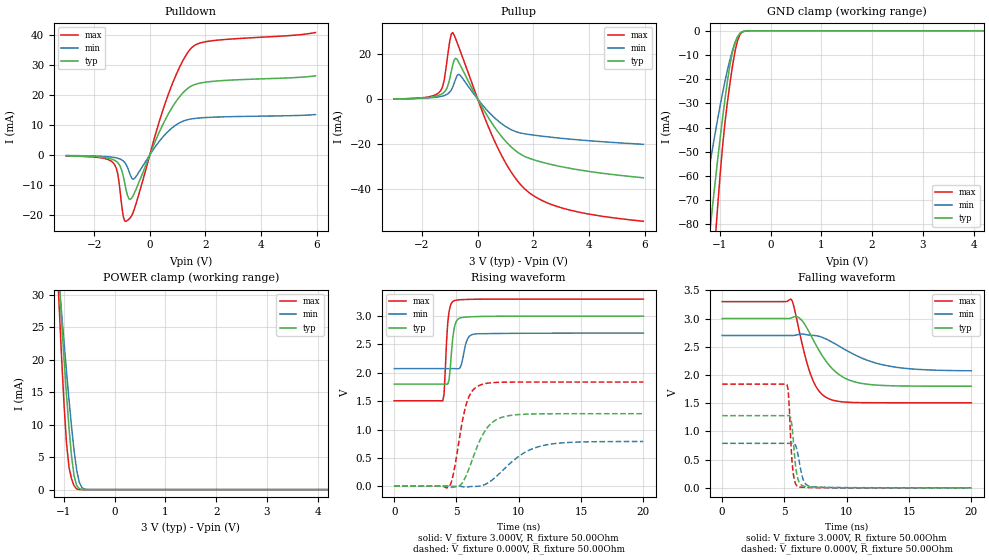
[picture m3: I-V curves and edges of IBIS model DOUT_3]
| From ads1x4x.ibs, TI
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|   DOutput 3.0V Model
[Model]   DOUT_3
Model_type   3-state
|Signals   DOUT_nDRDY
| variable   typ   min   max
|C_comp Output Tri-state
C_comp   3.796pF   4.715pF   2.919pF
|C_comp Output Low
|C_comp   7.402pF   8.505pF   5.981pF
|C_comp Output High
|C_comp   7.018pF   8.098pF   7.325pF
[Model Spec]
|Timing spec test load voltage corners 0.45*VCC
Vmeas   1.5V   1.35V   1.65V
Vref   1.5V   1.35V   1.65V
|Junction Temperature
[Temperature Range]   40.0   105.0   -40.0
[Voltage range]   5.0V   4.75V   5.25V
[Pullup reference]   3.0V   2.7V   3.3V
[power clamp reference]   3.0V   2.7V   3.3V
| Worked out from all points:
|   slope of the pulldown table from 0 to 0.45 V, typ, clamps not added: 45.9 ohm
|   slope of the pullup table from 0 to 0.45 V, typ, clamps not added: 47.3 ohm
|   GND clamp passes 1 mA (typ) near -0.60 V on its own axis
|   POWER clamp passes 1 mA (typ) near -0.76 V on its own axis
|   falling waveform, V_fixture 3.000V, R_fixture 50.00Ohm: 20-80 % time 2.2ns typ, 3.66ns min, 1.34ns max; typ from 3 V to 1.8 V
|   rising waveform, V_fixture 3.000V, R_fixture 50.00Ohm: 20-80 % time 313ps typ, 394ps min, 271ps max; typ from 1.8 V to 3 V
|   rising waveform, V_fixture 0.000V, R_fixture 50.00Ohm: 20-80 % time 1.53ns typ, 2.67ns min, 937ps max; typ from 0 V to 1.28 V
|   falling waveform, V_fixture 0.000V, R_fixture 50.00Ohm: 20-80 % time 344ps typ, 440ps min, 278ps max; typ from 1.28 V to 0 V
[Pulldown]
|   Voltage   I(typ)   I(min)   I(max)
-3V       -311.5uA   -207.5uA   -347.1uA
-1.3V     -1.667mA   -829.7uA   -2.805mA
-1.15V    -2.628mA   -1.121mA   -6.422mA
-1.05V    -4.09mA    -1.455mA   -13.56mA
-950mV    -7.253mA   -2.041mA   -20.69mA
-850mV    -11.75mA   -3.206mA   -22.19mA
-700mV    -14.86mA   -6.732mA   -21mA
-550mV    -12.68mA   -7.869mA   -17.94mA
600mV     12.56mA    7.307mA    18.53mA
1.1V      19.78mA    10.88mA    29.89mA
1.5V      23.06mA    12.03mA    35.79mA
5.95V     26.41mA    13.46mA    40.89mA
[GND Clamp]
|   Voltage   I(typ)   I(min)   I(max)
-3V       -488.9mA   -338.5mA   -693.5mA
-1.4V     -124.9mA   -82.22mA   -180.9mA
-1.35V    -114.4mA   -75.38mA   -165.2mA
-1.2V     -83.67mA   -55.66mA   -118.9mA
-1.15V    -73.79mA   -49.39mA   -103.9mA
-1.1V     -64.11mA   -43.29mA   -89.08mA
-1.05V    -54.69mA   -37.37mA   -74.73mA
-950mV    -36.78mA   -26.21mA   -48.68mA
-800mV    -14.07mA   -11.85mA   -21.67mA
-650mV    -2.397mA   -2.491mA   -3.953mA
-550mV    -339.5uA   -376.7uA   -400.6uA
5.95V     0A         0A         0A
[Pullup]
|   Voltage   I(typ)   I(min)   I(max)
-3V       89.08uA    85.18uA    74.35uA
-1.35V    1.903mA    1.112mA    3.478mA
-1.2V     3.138mA    1.59mA     8.716mA
-1.1V     5.057mA    2.151mA    17.41mA
-1V       9.308mA    3.18mA     26mA
-900mV    15.02mA    5.288mA    29.5mA
-800mV    18.11mA    8.719mA    26.98mA
-650mV    15.54mA    10.82mA    22.08mA
650mV     -13.17mA   -8.768mA   -19.77mA
1.65V     -25.17mA   -15.29mA   -39.32mA
3.1V      -30.17mA   -17.47mA   -48.49mA
5.95V     -34.86mA   -20.03mA   -54.14mA
[POWER Clamp]
|   Voltage   I(typ)   I(min)   I(max)
-3V       210.4mA    183.1mA    247.3mA
-1.1V     32.58mA    32.34mA    29.04mA
-1.05V    26.27mA    27.51mA    20.82mA
-1V       20.23mA    22.78mA    13.27mA
-950mV    14.56mA    18.18mA    7.113mA
-900mV    9.406mA    13.76mA    3.405mA
-850mV    5.07mA     9.617mA    1.627mA
-800mV    2.088mA    5.941mA    579.2uA
-750mV    647.5uA    3.017mA    107.9uA
-650mV    29.24uA    327.1uA    2.074uA
-550mV    1.126uA    18.06uA    52.24nA
5.95V     0A         0A         0A
[Ramp]
R_load = 50.00Ohm
|   typ   min   max
dV/dt_r   767.516mV/1.534ns   473.345mV/2.670ns   1.103V/936.808ps
dV/dt_f   719.578mV/2.204ns   375.497mV/3.656ns   1.076V/1.335ns
[Falling Waveform]
V_fixture = 3.000V
V_fixture_min = 2.700V
V_fixture_max = 3.300V
R_fixture = 50.00Ohm
|   Time   V(typ)   V(min)   V(max)
0s        3V         2.7V       3.3V
5.6ns     3.015V     2.7V       3.326V
6.3ns     2.99V      2.722V     2.669V
7.2ns     2.67V      2.703V     1.952V
7.8ns     2.427V     2.684V     1.709V
8.6ns     2.17V      2.609V     1.575V
9.8ns     1.95V      2.458V     1.521V
11.5ns    1.841V     2.274V     1.509V
14.6ns    1.805V     2.12V      1.508V
20ns      1.801V     2.074V     1.507V
[Rising Waveform]
V_fixture = 3.000V
V_fixture_min = 2.700V
V_fixture_max = 3.300V
R_fixture = 50.00Ohm
|   Time   V(typ)   V(min)   V(max)
0s        1.801V     2.074V     1.507V
3.9ns     1.801V     2.074V     1.507V
4ns       1.801V     2.074V     1.619V
4.3ns     1.803V     2.074V     2.886V
4.5ns     2.076V     2.074V     3.177V
4.8ns     2.768V     2.074V     3.27V
5.3ns     2.969V     2.094V     3.289V
5.8ns     2.984V     2.552V     3.294V
6.4ns     2.991V     2.683V     3.297V
20ns      3V         2.7V       3.3V
[Rising Waveform]
V_fixture = 0.000V
V_fixture_min = 0.000V
V_fixture_max = 0.000V
R_fixture = 50.00Ohm
|   Time   V(typ)   V(min)   V(max)
0s        793.8pV    878.1pV    783.1pV
4.4ns     -4.607mV   1.582uV    -8.19mV
4.7ns     -21.35mV   29.96uV    165.7mV
5.3ns     18.1mV     -1.994mV   930.7mV
5.8ns     198.9mV    -15.48mV   1.459V
6.2ns     426.9mV    -5.35mV    1.661V
6.9ns     818.2mV    3.927mV    1.784V
8.4ns     1.195V     213.5mV    1.833V
11.7ns    1.276V     704.1mV    1.838V
20ns      1.279V     788.9mV    1.838V
[Falling Waveform]
V_fixture = 0.000V
V_fixture_min = 0.000V
V_fixture_max = 0.000V
R_fixture = 50.00Ohm
|   Time   V(typ)   V(min)   V(max)
0s        1.279V     788.9mV    1.838V
5.2ns     1.28V      788.8mV    1.832V
5.3ns     1.281V     788.8mV    1.742V
5.5ns     1.246V     789.8mV    876.8mV
5.7ns     883.2mV    792.8mV    263.9mV
5.9ns     380.6mV    753.6mV    68.07mV
6.1ns     142.6mV    579mV      20.38mV
6.5ns     34.28mV    150.5mV    9.861mV
7.1ns     13.22mV    24.24mV    4.924mV
20ns      793.8pV    878.1pV    783.1pV
